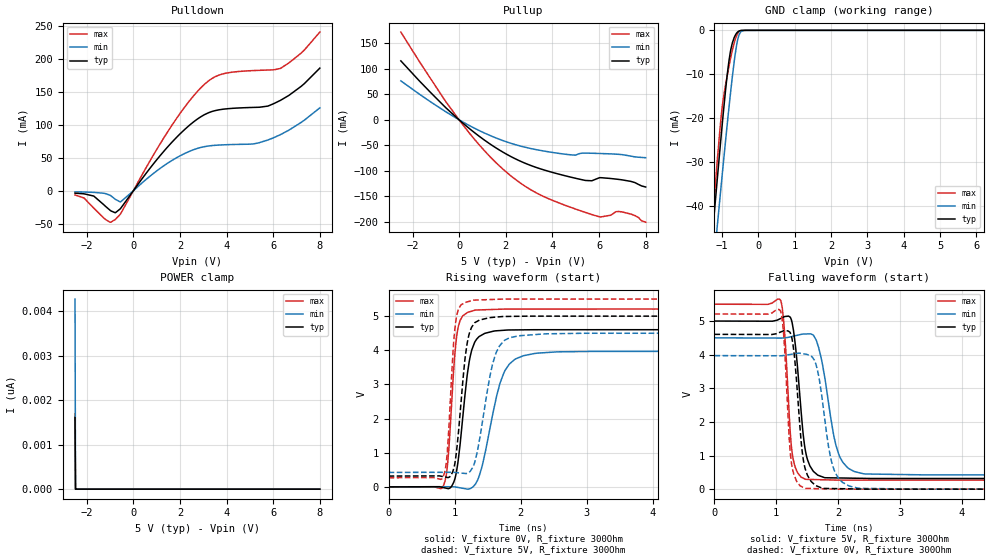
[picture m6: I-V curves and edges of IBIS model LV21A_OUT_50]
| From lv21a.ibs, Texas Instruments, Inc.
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|   Model LV21A_OUT_50
[Model]   LV21A_OUT_50
Model_type   Output
Polarity   Non-Inverting
Vmeas = 2.5
Vref = 0
Cref = 2pF
Rref = 100000
|   typ   min   max
C_comp   5.7pF   5.6pF   6pF
[Voltage Range]   5   4.5   5.5
[Temperature Range]   25   125   -40
[Pullup Reference]   5   4.5   5.5
[Pulldown Reference]   -0   0   0
[Power Clamp Reference]   5   4.5   5.5
[GND Clamp Reference]   0   0   0
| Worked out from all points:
|   slope of the pulldown table from 0 to 0.75 V, typ, clamps not added: 20.9 ohm
|   slope of the pullup table from 0 to 0.75 V, typ, clamps not added: 26.5 ohm
|   GND clamp passes 1 mA (typ) near -0.62 V on its own axis
|   falling waveform, V_fixture 5V, R_fixture 300Ohm: 20-80 % time 140ps typ, 226ps min, 99.7ps max; typ from 5 V to 0.317 V
|   rising waveform, V_fixture 0V, R_fixture 300Ohm: 20-80 % time 159ps typ, 276ps min, 108ps max; typ from 0 V to 4.6 V
|   rising waveform, V_fixture 5V, R_fixture 300Ohm: 20-80 % time 138ps typ, 225ps min, 95.8ps max; typ from 0.317 V to 5 V
|   falling waveform, V_fixture 0V, R_fixture 300Ohm: 20-80 % time 127ps typ, 194ps min, 93.3ps max; typ from 4.6 V to 0 V
[Pulldown]
|   Voltage   I(typ)   I(min)   I(max)
-2.5V     -3.475mA   -1.476mA   -6.196mA
-1.702V   -7.806mA   -2.267mA   -25.93mA
-998.5mV  -29.36mA   -6.592mA   -47.52mA
-778mV    -33.14mA   -12.61mA   -43.47mA
-547mV    -26.77mA   -16.75mA   -34.87mA
1.605V    71.87mA    45.02mA    96.8mA
3.034V    115.3mA    66.97mA    161.1mA
3.958V    124.3mA    69.99mA    178.4mA
5.28V     126.8mA    72.12mA    182.7mA
6.309V    137.3mA    85.34mA    185.7mA
7.191V    158.4mA    103.7mA    208.8mA
8V        186.3mA    126mA      240.9mA
[GND Clamp]
|   Voltage   I(typ)   I(min)   I(max)
-2.5V     -170.7mA   -168.9mA   -187.4mA
-1.282V   -49.09mA   -58.54mA   -46.61mA
-1.24V    -45.04mA   -54.83mA   -42.02mA
-1.208V   -42.02mA   -52.06mA   -38.61mA
-1.125V   -34.05mA   -44.71mA   -29.82mA
-977.5mV  -20.62mA   -32.07mA   -16.86mA
-799mV    -6.847mA   -17.4mA    -8.124mA
-715mV    -3.091mA   -11.05mA   -4.817mA
-641.5mV  -1.357mA   -6.134mA   -2.454mA
-526mV    -161.3uA   -1.092mA   -287.1uA
-379mV    -1.459uA   -24.15uA   -792nA
8V        0A         0A         0A
[Pullup]
|   Voltage   I(typ)   I(min)   I(max)
-2.5V     115.7mA    76.52mA    172.2mA
-641.5mV  27mA       17.92mA    40.48mA
282.5mV   -11.09mA   -7.276mA   -16.9mA
1.312V    -46.88mA   -30.36mA   -71.46mA
2.341V    -74.75mA   -47.61mA   -114.2mA
3.517V    -96.43mA   -60.13mA   -147.9mA
4.84V     -112.9mA   -68.8mA    -172.3mA
5.417V    -118.8mA   -65.15mA   -181.5mA
6.058V    -113.3mA   -65.95mA   -190.3mA
6.971V    -117.5mA   -68.06mA   -180.4mA
7.527V    -122.8mA   -72.47mA   -187.4mA
8V        -131.6mA   -74.18mA   -200.6mA
[POWER Clamp]
|   Voltage   I(typ)   I(min)   I(max)
-2.5V     1.613nA    4.273nA    1.697nA
-2.479V   0A         0A         0A
-2.469V   0A         0A         0A
8V        0A         0A         0A
[Ramp]
R_load = 300
|   typ   min   max
dV/dt_r   2.76245/1.58562e-10   2.38273/2.71866e-10   3.12538/1.07012e-10
dV/dt_f   2.80984/1.3974e-10   2.44575/2.24836e-10   3.13917/9.96818e-11
[Falling Waveform]
V_fixture = 5V
V_fixture_min = 4.5V
V_fixture_max = 5.5V
R_fixture = 300Ohm
C_fixture = 0F
|   Time   V(typ)   V(min)   V(max)
0s        5V         4.5V       5.5V
1.07ns    5.075V     4.494V     5.615V
1.132ns   5.13V      4.501V     4.714V
1.221ns   5.12V      4.527V     1.816V
1.257ns   4.945V     4.542V     1.072V
1.47ns    1.148V     4.615V     294.2mV
1.685ns   407.1mV    4.207V     282.6mV
2.021ns   333mV      988.1mV    268.3mV
2.406ns   321.6mV    458.4mV    268.3mV
15ns      316.9mV    423.7mV    268mV
[Rising Waveform]
V_fixture = 0V
V_fixture_min = 0V
V_fixture_max = 0V
R_fixture = 300Ohm
C_fixture = 0F
|   Time   V(typ)   V(min)   V(max)
0s        9.962uV    7.308uV    10.41uV
826ps     -18.73mV   4.01mV     13.47mV
894.1ps   -47.83mV   4.34mV     708.6mV
996.4ps   197.9mV    1.92mV     3.754V
1.045ns   660.1mV    -13.99mV   4.596V
1.193ns   3.332V     -65.76mV   5.105V
1.309ns   4.257V     70.38mV    5.176V
1.744ns   4.586V     3.342V     5.206V
2.203ns   4.602V     3.904V     5.207V
15ns      4.604V     3.971V     5.209V
[Rising Waveform]
V_fixture = 5V
V_fixture_min = 4.5V
V_fixture_max = 5.5V
R_fixture = 300Ohm
C_fixture = 0F
|   Time   V(typ)   V(min)   V(max)
0s        316.9mV    423.7mV    268mV
823.8ps   300.6mV    426.7mV    283.9mV
882.6ps   277.5mV    426.9mV    901.1mV
975.8ps   479.5mV    425.7mV    3.999V
1.025ns   1.009V     418.5mV    4.959V
1.158ns   3.783V     392.8mV    5.4V
1.283ns   4.75V      610.2mV    5.466V
1.615ns   4.97V      3.87V      5.491V
1.964ns   4.996V     4.422V     5.5V
15ns      5V         4.5V       5.5V
[Falling Waveform]
|Gnd
V_fixture = 0V
V_fixture_min = 0V
V_fixture_max = 0V
R_fixture = 300Ohm
C_fixture = 0F
|   Time   V(typ)   V(min)   V(max)
0s        4.604V     3.971V     5.209V
1.064ns   4.67V      3.967V     5.311V
1.125ns   4.715V     3.978V     4.458V
1.206ns   4.686V     4.001V     1.584V
1.243ns   4.554V     4.011V     800.8mV
1.462ns   640.3mV    4.018V     24.63mV
1.661ns   89.4mV     3.573V     14.51mV
1.935ns   17.48mV    571.2mV    3.291mV
2.318ns   5.665mV    30.93mV    275.8uV
15ns      10.19uV    8.433uV    12.55uV
